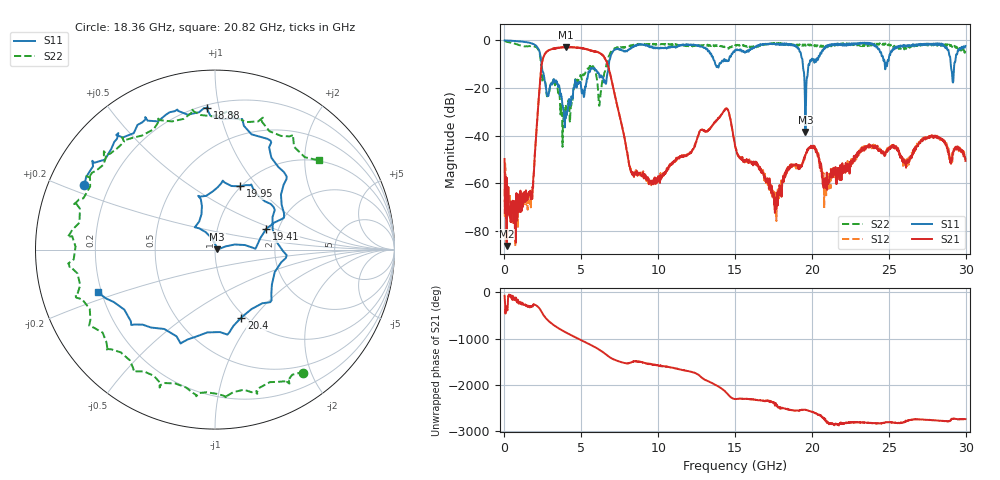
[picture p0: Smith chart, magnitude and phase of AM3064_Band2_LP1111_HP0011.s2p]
# Hz S DB R 50.0
!freq dBS11 angS11 dBS21 angS21 dBS12 angS12 dBS22 angS22
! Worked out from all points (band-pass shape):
!   1600 points, 10 MHz to 29.98 GHz, reference 50 ohm
!   highest |S21| = -2.72 dB at 4.002 GHz (marker M1); lowest = -86.3 dB at 141.2 MHz (marker M2)
!   |S21| within 3 dB of the highest: 2.627 GHz to 6.288 GHz (3.662 GHz wide, 82.1 % of centre); 6.291508 GHz to 6.309476 GHz (17.97 MHz wide, 0.285 % of centre)
!   lowest |S11| = -38.4 dB at 19.58 GHz (marker M3), VSWR 1.02, Z = 51.2 + j0.228 ohm
!   |S11| at or under -10 dB: 2.413 GHz to 6.786 GHz (4.372 GHz wide, 95.1 % of centre); 13.72 GHz to 13.98 GHz (257.6 MHz wide, 1.86 % of centre); 19.41 GHz to 19.83 GHz (426.7 MHz wide, 2.17 % of centre)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
!   |S22| runs from -44.6 to -0.1 dB; largest |S21 - S12| = 0.025
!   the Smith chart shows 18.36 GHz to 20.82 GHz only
!   S11 on the Smith chart (normalised r, x): 18.36 GHz: 0.11, +0.23; 18.88 GHz: 0.22, +0.92; 19.41 GHz: 1.73, +0.44; 19.95 GHz: 0.99, +0.82; 20.4 GHz: 0.96, -0.87; 20.82 GHz: 0.19, -0.17
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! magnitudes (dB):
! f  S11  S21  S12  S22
! 10 MHz  0.0  -49.7  -62.3  -0.1
! 141.2 MHz  0.0  -86.3  -67.2  -0.5
! 1.697 GHz  -1.1  -64.0  -64.2  -2.4
! 2.522 GHz  -13.5  -7.3  -7.2  -15.5
! 4.002 GHz  -29.8  -2.7  -2.8  -27.7
! 5.015 GHz  -21.4  -3.3  -3.2  -15.9
! 6.627 GHz  -17.3  -8.8  -8.8  -10.2
! 8.276 GHz  -2.9  -55.7  -55.7  -2.1
! 10 GHz  -3.3  -56.9  -58.2  -1.7
! 14.39 GHz  -8.6  -28.8  -28.8  -3.2
! 15 GHz  -4.2  -44.3  -44.4  -2.1
! 17.61 GHz  -1.5  -66.6  -66.2  -1.0
! 18.36 GHz  -1.8  -55.0  -53.7  -1.5
! 18.88 GHz  -2.0  -52.3  -52.9  -2.2
! 19.41 GHz  -10.2  -51.2  -51.2  -1.7
! 19.58 GHz  -38.4  -48.0  -47.9  -2.1
! 19.95 GHz  -8.4  -44.8  -44.6  -2.1
! 19.99 GHz  -7.8  -44.9  -44.6  -1.7
! 20.4 GHz  -7.8  -48.0  -47.2  -2.5
! 20.82 GHz  -3.2  -59.3  -60.9  -2.3
! 25 GHz  -7.9  -45.2  -45.0  -1.6
! 29.98 GHz  -2.3  -50.5  -49.9  -4.4
